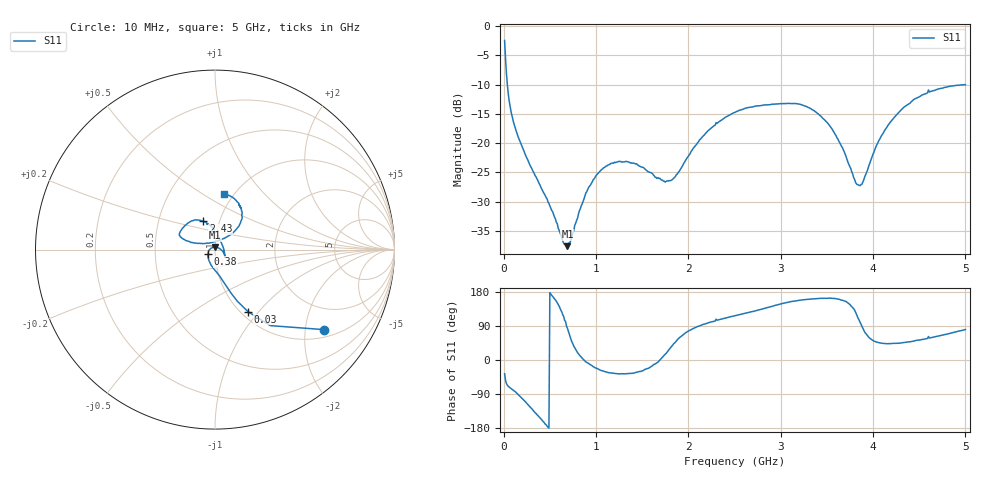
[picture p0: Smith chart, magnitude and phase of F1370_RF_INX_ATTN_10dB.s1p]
! S-parameters for RF_INX input IDT F1370 DPD Demodulator
! Date Measured:  2015-11-25  RGG
!  Port 1 = Pin 35 = RF_INX
! STATE: RF_INX selected, 10 dB attenuation (Gain = Gmax - 10 dB)
! RF Frequency:  10 MHz to 5000 MHz
! RF_INY, IF_I+, IF_I-, IF_Q+, and IF_Q- terminated
! 2300 MHz, 0 dBm signal applied to LO_IN
! Vcc = +5.00 Volts  Icc = approx 275 mA.
! NOTES:  The device was measured on a custom printed circuit evaluation board with individual 50 ohm
!  microstrip lines to the RF and LO pins. The 50 ohm microstrip lines were de-embedded using reference
!  plane extensions
! Instrument Manufacturer:  Agilent Technologies
! Instrument Model:  E5071C
! Instrument Serial Number:  MY46419053
! Instrument Firmware Rev:  A.11.31
! Frequency Re{S11} Im{S11}
# HZ  S  RI R 50.00
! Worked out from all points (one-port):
!   500 points, 10 MHz to 5 GHz, reference 50 ohm
!   lowest |S11| = -37.6 dB at 690 MHz (marker M1), VSWR 1.03, Z = 50.1 + j1.31 ohm
!   |S11| at or under -10 dB: 39.49 MHz to end of sweep
!   S11 on the Smith chart (normalised r, x): 10 MHz: 1.23, -2.52; 30 MHz: 1.08, -0.88; 380 MHz: 0.92, -0.04; 2.43 GHz: 0.84, +0.27; 5 GHz: 0.91, +0.62
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1e7  0.6063 -0.4458
3e7  0.1831 -0.3451
4e7  0.124 -0.2871
6e7  0.0719 -0.2162
1.2e8  0.0175 -0.1373
3.8e8  -0.0392 -0.0235
6.4e8  -0.00709 0.0127
6.9e8  0.00141 0.0131
9e8  0.0381 -0.00425
9.8e8  0.0467 -0.016
1.26e9  0.0558 -0.0413
1.43e9  0.0554 -0.0361
1.74e9  0.046 0.0104
1.89e9  0.0315 0.0465
2.14e9  -0.00385 0.11
2.43e9  -0.0655 0.1576
2.51e9  -0.0838 0.1632
3.13e9  -0.1965 0.0925
3.33e9  -0.1844 0.064
3.5e9  -0.1438 0.0451
3.66e9  -0.0866 0.035
3.76e9  -0.0481 0.0361
3.82e9  -0.023 0.0384
3.87e9  -0.00269 0.0441
4.11e9  0.0873 0.0842
4.38e9  0.1435 0.1584
4.62e9  0.144 0.2348
5e9  0.0528 0.3101
